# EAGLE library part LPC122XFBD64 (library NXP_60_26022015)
NXP ARM M0 32 bit Microcontroller AAL Eindhoven MV+ MK
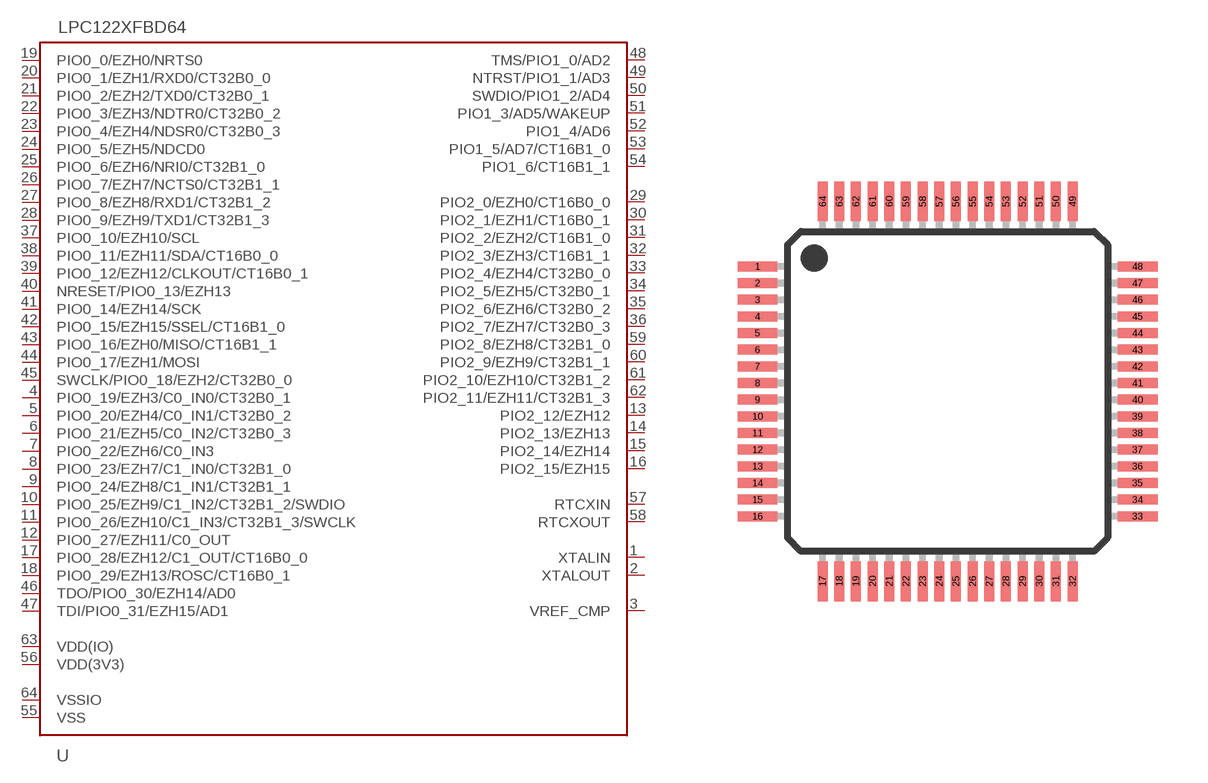
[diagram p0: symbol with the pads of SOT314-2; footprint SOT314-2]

Designator prefix U

## LPC122XFBD64  [SOT314-2]
1  XTALIN
2  XTALOUT
3  VREF_CMP
4  PIO0_19/EZH3/C0_IN0/CT32B0_1
5  PIO0_20/EZH4/C0_IN1/CT32B0_2
6  PIO0_21/EZH5/C0_IN2/CT32B0_3
7  PIO0_22/EZH6/C0_IN3
8  PIO0_23/EZH7/C1_IN0/CT32B1_0
9  PIO0_24/EZH8/C1_IN1/CT32B1_1
10  PIO0_25/EZH9/C1_IN2/CT32B1_2/SWDIO
11  PIO0_26/EZH10/C1_IN3/CT32B1_3/SWCLK
12  PIO0_27/EZH11/C0_OUT
13  PIO2_12/EZH12
14  PIO2_13/EZH13
15  PIO2_14/EZH14
16  PIO2_15/EZH15
17  PIO0_28/EZH12/C1_OUT/CT16B0_0
18  PIO0_29/EZH13/ROSC/CT16B0_1
19  PIO0_0/EZH0/NRTS0
20  PIO0_1/EZH1/RXD0/CT32B0_0
21  PIO0_2/EZH2/TXD0/CT32B0_1
22  PIO0_3/EZH3/NDTR0/CT32B0_2
23  PIO0_4/EZH4/NDSR0/CT32B0_3
24  PIO0_5/EZH5/NDCD0
25  PIO0_6/EZH6/NRI0/CT32B1_0
26  PIO0_7/EZH7/NCTS0/CT32B1_1
27  PIO0_8/EZH8/RXD1/CT32B1_2
28  PIO0_9/EZH9/TXD1/CT32B1_3
29  PIO2_0/EZH0/CT16B0_0
30  PIO2_1/EZH1/CT16B0_1
31  PIO2_2/EZH2/CT16B1_0
32  PIO2_3/EZH3/CT16B1_1
33  PIO2_4/EZH4/CT32B0_0
34  PIO2_5/EZH5/CT32B0_1
35  PIO2_6/EZH6/CT32B0_2
36  PIO2_7/EZH7/CT32B0_3
37  PIO0_10/EZH10/SCL
38  PIO0_11/EZH11/SDA/CT16B0_0
39  PIO0_12/EZH12/CLKOUT/CT16B0_1
40  NRESET/PIO0_13/EZH13
41  PIO0_14/EZH14/SCK
42  PIO0_15/EZH15/SSEL/CT16B1_0
43  PIO0_16/EZH0/MISO/CT16B1_1
44  PIO0_17/EZH1/MOSI
45  SWCLK/PIO0_18/EZH2/CT32B0_0
46  TDO/PIO0_30/EZH14/AD0
47  TDI/PIO0_31/EZH15/AD1
48  TMS/PIO1_0/AD2
49  NTRST/PIO1_1/AD3
50  SWDIO/PIO1_2/AD4
51  PIO1_3/AD5/WAKEUP
52  PIO1_4/AD6
53  PIO1_5/AD7/CT16B1_0
54  PIO1_6/CT16B1_1
55  VSS  pwr
56  VDD(3V3)  pwr
57  RTCXIN
58  RTCXOUT
59  PIO2_8/EZH8/CT32B1_0
60  PIO2_9/EZH9/CT32B1_1
61  PIO2_10/EZH10/CT32B1_2
62  PIO2_11/EZH11/CT32B1_3
63  VDD(IO)  pwr
64  VSSIO  pwr

## Footprint SOT314-2 (pad centres in mm)
SOT314-2 LQFP64: plastic low profile quad flat package; 64 leads; body 10 x 10 x 1.4 mm JEDEC: MS-026 IEC: 136E10
smd 1.2 x 0.3: 1 -5.7,3.75; 2 -5.7,3.25; 3 -5.7,2.75; 4 -5.7,2.25; 5 -5.7,1.75; 6 -5.7,1.25; 7 -5.7,0.75; 8 -5.7,0.25; 9 -5.7,-0.25; 10 -5.7,-0.75; 11 -5.7,-1.25; 12 -5.7,-1.75; 13 -5.7,-2.25; 14 -5.7,-2.75; 15 -5.7,-3.25; 16 -5.7,-3.75; 33 5.7,-3.75; 34 5.7,-3.25; 35 5.7,-2.75; 36 5.7,-2.25; 37 5.7,-1.75; 38 5.7,-1.25; 39 5.7,-0.75; 40 5.7,-0.25; 41 5.7,0.25; 42 5.7,0.75; 43 5.7,1.25; 44 5.7,1.75; 45 5.7,2.25; 46 5.7,2.75; 47 5.7,3.25; 48 5.7,3.75
smd 0.3 x 1.2: 17 -3.75,-5.7; 18 -3.25,-5.7; 19 -2.75,-5.7; 20 -2.25,-5.7; 21 -1.75,-5.7; 22 -1.25,-5.7; 23 -0.75,-5.7; 24 -0.25,-5.7; 25 0.25,-5.7; 26 0.75,-5.7; 27 1.25,-5.7; 28 1.75,-5.7; 29 2.25,-5.7; 30 2.75,-5.7; 31 3.25,-5.7; 32 3.75,-5.7; 49 3.75,5.7; 50 3.25,5.7; 51 2.75,5.7; 52 2.25,5.7; 53 1.75,5.7; 54 1.25,5.7; 55 0.75,5.7; 56 0.25,5.7; 57 -0.25,5.7; 58 -0.75,5.7; 59 -1.25,5.7; 60 -1.75,5.7; 61 -2.25,5.7; 62 -2.75,5.7; 63 -3.25,5.7; 64 -3.75,5.7

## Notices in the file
This library may be distributed and adapted freely for any purpose, as long as NXP is credited and any new creation is licensed under the same terms.
